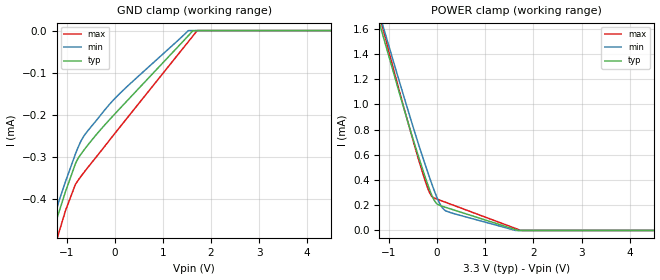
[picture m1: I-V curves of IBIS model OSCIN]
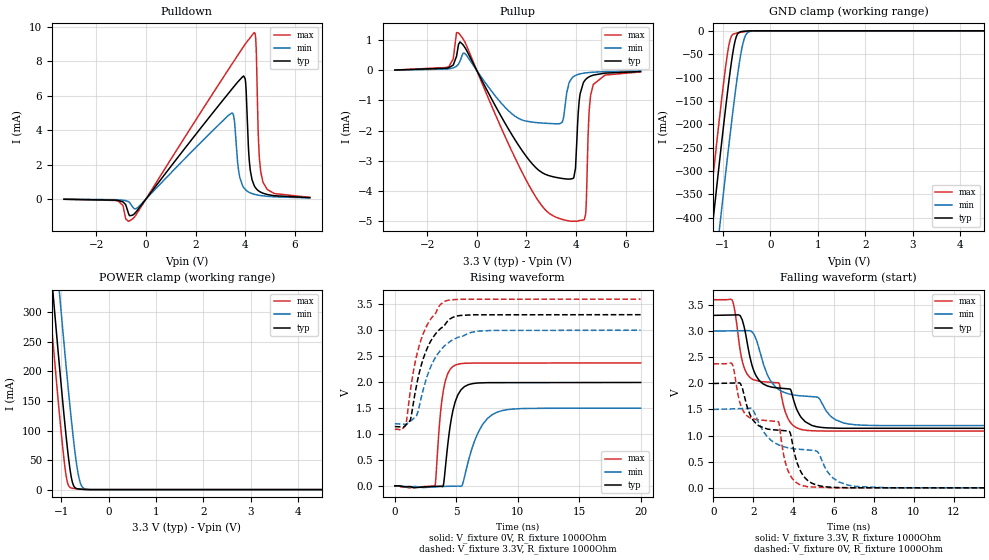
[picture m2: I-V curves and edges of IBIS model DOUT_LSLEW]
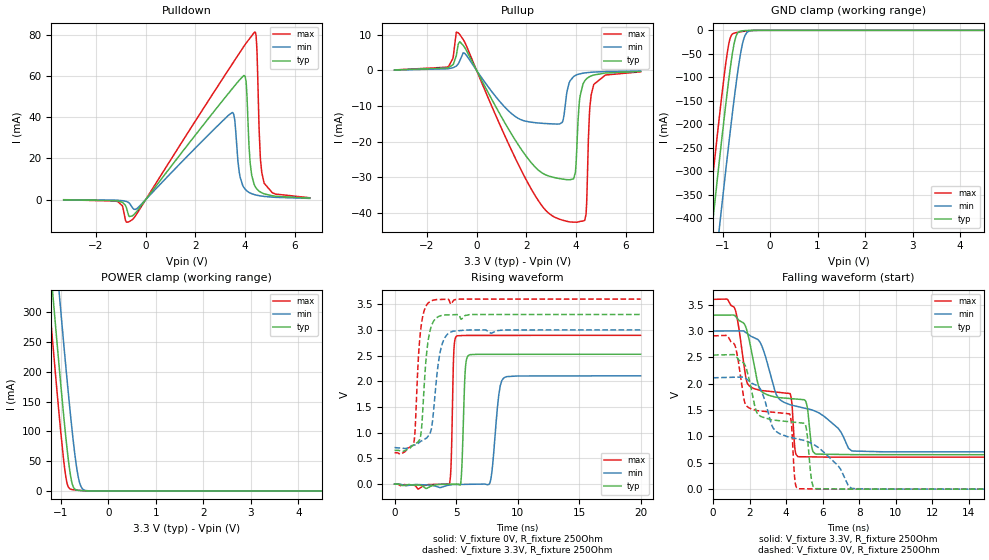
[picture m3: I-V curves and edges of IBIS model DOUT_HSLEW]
| Texas Instruments Incorporated
| LMX2615-SP Space Grade 40 MHz to 15 GHz Wideband Synthesizer with Phase
| Synchronization and JESD204B Support
[IBIS Ver]   4.1
[File name]   lmx2615.ibs
[File Rev]   1.0
[Date]   05/04/2018
[Source]   Model built from spectre simulations at:
   Texas Instruments Incorporated.
   Analog-eLab, HPA
   12500 TI Blvd
   Dallas, TX -75243
[Notes]   Revision History
| - Rev 1.0: 05/04/2018
| - C_comp although listed in numerical order of value are
|   obtained from varying PVT conditions. For PVT conditions for
|   each specific value refer the buffer description under
|   respective [Model]. IBIS model user is responsible for using
|   appropriate C_comp to simulate for Signal Integrity.
| - Notes regarding non-monotonicity of various models
|   have been reviewed and considered minor and can be ignored.
[Disclaimer]
| This model is designed as an aid for customers of Texas Instruments.
| TI and its licensors and suppliers make no warranties, either expressed
| or implied, with respect to this  model, including the warranties of
| merchantability or fitness for a particular purpose. The model is
| provided solely on an "as is" basis. The entire risk as to its quality
| and performance is with the customer.
| This model is subject to change without notice. Texas Instruments
| Incorporated is not responsible for updating this model.
[Copyright]
(C) Copyright 2018 Texas Instruments Incorporated.All rights reserved.
|  Component LMX2615W-MPR 64 pin CQFP Package
|  Part # LMX2615W-MPR
[Component]   LMX2615W-MPR
[Manufacturer]  TI
[Package]   | 64 pin CQFP Package
|   typ   min   max
R_pkg   0.05   0.04   0.06
L_pkg   1.0nH   0.8nH   1.2nH
C_pkg   0.2pF   0.16pF   0.24pF
[Pin]   signal_name   model_name   R_pin   L_pin   C_pin
1   NC   NC   NA   NA   NA
2   NC   NC   NA   NA   NA
3   FS0   INPCE   NA   NA   NA
4   FS1   INPCE   NA   NA   NA
5   CAL   INPCE   NA   NA   NA
6   GND   GND   NA   NA   NA
7   VbiasVCO   NC   NA   NA   NA
8   GND   GND   NA   NA   NA
9   NC   NC   NA   NA   NA
10   GND   GND   NA   NA   NA
11   VCCdig   POWER   NA   NA   NA
12   OSCinP   OSCIN   NA   NA   NA
13   OSCinM   OSCIN   NA   NA   NA
14   VregIN   NC   NA   NA   NA
15   FS2   INPCE   NA   NA   NA
16   FS3   INPCE   NA   NA   NA
17   FS4   INPCE   NA   NA   NA
18   FS5   INPCE   NA   NA   NA
19   FS6   INPCE   NA   NA   NA
20   FS7   INPCE   NA   NA   NA
21   VCCCP   POWER   NA   NA   NA
22   CPOUT   NC   NA   NA   NA
23   GND   GND   NA   NA   NA
24   GND   GND   NA   NA   NA
25   VCCMASH   POWER   NA   NA   NA
26   SCK   INP   NA   NA   NA
27   SDI   INP   NA   NA   NA
28   GND   GND   NA   NA   NA
29   RFOUTBM   RFOUT   NA   NA   NA
30   RFOUTBP   RFOUT   NA   NA   NA
31   GND   GND   NA   NA   NA
32   MUXOUT   DOUT   NA   NA   NA
33   NC   NC   NA   NA   NA
34   VCCBUF   POWER   NA   NA   NA
35   GND   GND   NA   NA   NA
36   RFOUTAM   RFOUT   NA   NA   NA
37   RFOUTAP   RFOUT   NA   NA   NA
38   GND   GND   NA   NA   NA
39   CSB   INP   NA   NA   NA
40   GND   GND   NA   NA   NA
41   VccVCO2   NC   NA   NA   NA
42   VbiasVCO2   NC   NA   NA   NA
43   NC   NC   NA   NA   NA
44   VrefVCO2   NC   NA   NA   NA
45   RECAL_EN   INP   NA   NA   NA
46   NC   NC   NA   NA   NA
47   NC   NC   NA   NA   NA
48   NC   NC   NA   NA   NA
49   NC   NC   NA   NA   NA
50   NC   NC   NA   NA   NA
51   GND   GND   NA   NA   NA
52   NC   NC   NA   NA   NA
53   VbiasVARAC   NC   NA   NA   NA
54   GND   GND   NA   NA   NA
55   Vtune   NC   NA   NA   NA
56   VREFVCO   NC   NA   NA   NA
57   VccVCO   NC   NA   NA   NA
58   NC   NC   NA   NA   NA
59   VregVCO   NC   NA   NA   NA
60   GND   GND   NA   NA   NA
61   GND   GND   NA   NA   NA
62   NC   NC   NA   NA   NA
63   NC   NC   NA   NA   NA
64   NC   NC   NA   NA   NA
[Diff pin]  inv_pin  vdiff  tdelay_typ  tdelay_min  tdelay_max
 12   13   0.1   NA   NA   NA
 30   29   NA   0.0s   0.0s   0.0s
 37   36   NA   0.0s   0.0s   0.0s
|  Component LMX2615W-MLS 64 pin CQFP Package
|  Part # LMX2615W-MLS
[Component]   LMX2615W-MLS
[Manufacturer]  TI
[Package]   | 64 pin CQFP Package
|   typ   min   max
R_pkg   0   0   0
L_pkg   0   0   0
C_pkg   0   0   0
[Pin]   signal_name   model_name   R_pin   L_pin   C_pin
1   NC   NC   NA   NA   NA
2   NC   NC   NA   NA   NA
3   FS0   INPCE   NA   NA   NA
4   FS1   INPCE   NA   NA   NA
5   CAL   INPCE   NA   NA   NA
6   GND   GND   NA   NA   NA
7   VbiasVCO   NC   NA   NA   NA
8   GND   GND   NA   NA   NA
9   NC   NC   NA   NA   NA
10   GND   GND   NA   NA   NA
11   VCCdig   POWER   NA   NA   NA
12   OSCinP   OSCIN   NA   NA   NA
13   OSCinM   OSCIN   NA   NA   NA
14   VregIN   NC   NA   NA   NA
15   FS2   INPCE   NA   NA   NA
16   FS3   INPCE   NA   NA   NA
17   FS4   INPCE   NA   NA   NA
18   FS5   INPCE   NA   NA   NA
19   FS6   INPCE   NA   NA   NA
20   FS7   INPCE   NA   NA   NA
21   VCCCP   POWER   NA   NA   NA
22   CPOUT   NC   NA   NA   NA
23   GND   GND   NA   NA   NA
24   GND   GND   NA   NA   NA
25   VCCMASH   POWER   NA   NA   NA
26   SCK   INP   NA   NA   NA
27   SDI   INP   NA   NA   NA
28   GND   GND   NA   NA   NA
29   RFOUTBM   RFOUT   NA   NA   NA
30   RFOUTBP   RFOUT   NA   NA   NA
31   GND   GND   NA   NA   NA
32   MUXOUT   DOUT   NA   NA   NA
33   NC   NC   NA   NA   NA
34   VCCBUF   POWER   NA   NA   NA
35   GND   GND   NA   NA   NA
36   RFOUTAM   RFOUT   NA   NA   NA
37   RFOUTAP   RFOUT   NA   NA   NA
38   GND   GND   NA   NA   NA
39   CSB   INP   NA   NA   NA
40   GND   GND   NA   NA   NA
41   VccVCO2   NC   NA   NA   NA
42   VbiasVCO2   NC   NA   NA   NA
43   NC   NC   NA   NA   NA
44   VrefVCO2   NC   NA   NA   NA
45   RECAL_EN   INP   NA   NA   NA
46   NC   NC   NA   NA   NA
47   NC   NC   NA   NA   NA
48   NC   NC   NA   NA   NA
49   NC   NC   NA   NA   NA
50   NC   NC   NA   NA   NA
51   GND   GND   NA   NA   NA
52   NC   NC   NA   NA   NA
53   VbiasVARAC   NC   NA   NA   NA
54   GND   GND   NA   NA   NA
55   Vtune   NC   NA   NA   NA
56   VREFVCO   NC   NA   NA   NA
57   VccVCO   NC   NA   NA   NA
58   NC   NC   NA   NA   NA
59   VregVCO   NC   NA   NA   NA
60   GND   GND   NA   NA   NA
61   GND   GND   NA   NA   NA
62   NC   NC   NA   NA   NA
63   NC   NC   NA   NA   NA
64   NC   NC   NA   NA   NA
[Diff pin]  inv_pin  vdiff  tdelay_typ  tdelay_min  tdelay_max
 12   13   0.1   NA   NA   NA
 30   29   NA   0.0s   0.0s   0.0s
 37   36   NA   0.0s   0.0s   0.0s
|   Model Selectors
[Model Selector] DOUT
DOUT_LSLEW   3.3V OUTPUT, low slew rate
DOUT_HSLEW   3.3V OUTPUT, high slew rate
| Models and submodels in the file (6): OSCIN (Input), DOUT_LSLEW (3-state), DOUT_HSLEW (3-state), INP (Input), INPCE (Input), RFOUT (Open_drain)
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|   Model OSCIN
[Model]   OSCIN
Model_type   Input
Vinl = .4
Vinh = 1.8
|   typ   min   max
C_comp   0.219p   0.215p   0.221p
[Voltage Range]   3.3   3.15   3.45
[Temperature Range]   27   125   -40
[Power Clamp Reference]   3.3   3.15   3.45
[GND Clamp Reference]   0   0   0
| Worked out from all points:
|   GND clamp passes 1 mA (typ) near -2.28 V on its own axis
|   POWER clamp passes 1 mA (typ) near -0.72 V on its own axis
[GND Clamp]
|   Voltage   I(typ)   I(min)   I(max)
-3.3V     -1.834mA   -1.951mA   -1.829mA
-1.508V   -565uA     -564.9uA   -620uA
-1.31V    -487.7uA   -467.1uA   -540.3uA
-1.152V   -429.5uA   -403.3uA   -477.7uA
-1.023V   -383.4uA   -359.6uA   -428.6uA
-815.1mV  -316.6uA   -293.4uA   -365.7uA
-607.2mV  -279.5uA   -245.5uA   -332.8uA
85.8mV    -188.1uA   -152.1uA   -232.8uA
1.531V    -12.08uA   -44.6nA    -26.36uA
1.62V     -735.5nA   0A         -13.62uA
1.729V    0A         0A         0A
6.6V      0A         0A         0A
[POWER Clamp]
|   Voltage   I(typ)   I(min)   I(max)
-3.3V     5.966mA    6.361mA    6.077mA
-1.231V   1.684mA    1.757mA    1.748mA
-815.1mV  1.129mA    1.218mA    1.146mA
-409.2mV  611.5uA    709.5uA    592.2uA
-181.5mV  349.1uA    446uA      320.6uA
-112.2mV  280.1uA    369.9uA    271.2uA
-23.1mV   218uA      278.7uA    251.5uA
105.6mV   191.7uA    180.2uA    233.1uA
184.8mV   182uA      154.2uA    221.8uA
1.63V     6.809uA    0A         15.72uA
1.729V    0A         0A         1.069uA
6.6V      0A         0A         0A
|   Model DOUT_LSLEW
[Model]   DOUT_LSLEW
Model_type   3-state
Polarity   Non-Inverting
Vmeas = 1.65
Vref = 3.3
Cref = 1pF
Rref = 1000
|   typ   min   max
|   (nom PVT)   (fast PVT)   (slow PVT)
C_comp   1.019p   0.968p   1.051p
[Voltage Range]   3.3   3   3.6
[Temperature Range]   27   125   -40
[Pullup Reference]   3.3   3   3.6
[Pulldown Reference]   0   0   0
[Power Clamp Reference]   3.3   3   3.6
[GND Clamp Reference]   0   0   0
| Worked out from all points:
|   slope of the pulldown table from 0 to 0.495 V, typ, clamps not added: 528 ohm
|   slope of the pullup table from 0 to 0.495 V, typ, clamps not added: 627 ohm
|   GND clamp passes 1 mA (typ) near -0.57 V on its own axis
|   POWER clamp passes 1 mA (typ) near -0.63 V on its own axis
|   falling waveform, V_fixture 3.3V, R_fixture 1000Ohm: 20-80 % time 2.45ns typ, 3.22ns min, 2.31ns max; typ from 3.3 V to 1.14 V
|   rising waveform, V_fixture 0V, R_fixture 1000Ohm: 20-80 % time 749ps typ, 1.4ns min, 569ps max; typ from 0 V to 1.99 V
|   rising waveform, V_fixture 3.3V, R_fixture 1000Ohm: 20-80 % time 1.63ns typ, 1.79ns min, 1.49ns max; typ from 1.14 V to 3.3 V
|   falling waveform, V_fixture 0V, R_fixture 1000Ohm: 20-80 % time 2.61ns typ, 3.39ns min, 2.43ns max; typ from 2 V to 0 V
[Pulldown]
|   Voltage   I(typ)   I(min)   I(max)
-3.3V     -11.43uA   -7.802uA   -12.1uA
-537.9mV  -936.6uA   -451.7uA   -1.153mA
3.462V    6.382mA    4.997mA    7.828mA
3.759V    6.891mA    1.418mA    8.479mA
3.937V    7.142mA    671.1uA    8.867mA
4.016V    6.747mA    535.7uA    9.031mA
4.165V    2.21mA     385.6uA    9.304mA
4.372V    751.3uA    275.1uA    9.665mA
4.442V    605.9uA    250.9uA    8.713mA
4.561V    452.6uA    217.8uA    2.597mA
4.709V    342.4uA    186.9uA    1.005mA
6.6V      81.82uA    66.05uA    100.7uA
[GND Clamp]
|   Voltage   I(typ)   I(min)   I(max)
-3.3V     -2.452A    -2.589A    -2.364A
-1.439V   -627.2mA   -770.9mA   -533mA
-1.27V    -466.7mA   -610.7mA   -372.2mA
-1.211V   -410.7mA   -554.6mA   -316.2mA
-1.073V   -282mA     -425.3mA   -188.4mA
-1.033V   -246mA     -388.8mA   -153.2mA
-874.5mV  -109.2mA   -246.3mA   -31.62mA
-765.6mV  -33.07mA   -153.9mA   -6.398mA
-696.3mV  -7.92mA    -99.78mA   -4.642mA
-577.5mV  -1.073mA   -27.36mA   -2.516mA
-419.1mV  -88.15uA   -1.084mA   -769.1uA
6.6V      0A         0A         0A
[Pullup]
|   Voltage   I(typ)   I(min)   I(max)
-3.3V     12.07uA    9.347uA    12.51uA
-1.132V   89.8uA     52.94uA    125.7uA
-735.9mV  862.4uA    206.3uA    1.249mA
2.234V    -3.109mA   -1.72mA    -4.015mA
3.432V    -3.594mA   -1.729mA   -4.955mA
3.858V    -3.601mA   -234.1uA   -5.021mA
3.977V    -3.257mA   -167uA     -5.022mA
4.145V    -883.9uA   -117.5uA   -4.995mA
4.382V    -304.1uA   -82.23uA   -4.8mA
4.521V    -215.1uA   -69.84uA   -1.435mA
4.699V    -155.4uA   -58.43uA   -464.3uA
6.6V      -38.28uA   -21.08uA   -49.46uA
[POWER Clamp]
|   Voltage   I(typ)   I(min)   I(max)
-3.3V     2.408A     2.526A     2.331A
-1.389V   536.7mA    662mA      454.1mA
-1.231V   386.9mA    512.5mA    303.9mA
-1.171V   331.5mA    457.1mA    248.6mA
-1.053V   223.1mA    347.7mA    141.4mA
-1.013V   188mA      311.9mA    107.5mA
-894.3mV  88.96mA    207.3mA    22.7mA
-795.3mV  24.72mA    125.6mA    2.896mA
-735.9mV  6.329mA    81.34mA    1.968mA
-636.9mV  1.065mA    24.47mA    1.107mA
-478.5mV  181.4uA    709.5uA    176.1uA
6.6V      0A         0A         0A
[Ramp]
R_load = 1000
|   typ   min   max
dV/dt_r   1.19558/7.49454e-10   0.89825/1.40115e-09   1.4217/5.69081e-10
dV/dt_f   1.29663/2.44804e-09   1.08511/3.20365e-09   1.50804/2.31143e-09
[Falling Waveform]
V_fixture = 3.3V
V_fixture_min = 3V
V_fixture_max = 3.6V
R_fixture = 1000Ohm
C_fixture = 0F
|   Time   V(typ)   V(min)   V(max)
0s        3.3V       3V         3.6V
928.8ps   3.307V     3.005V     3.597V
1.34ns    3.295V     3.007V     2.629V
1.669ns   2.822V     3.008V     2.186V
2.149ns   2.133V     2.83V      2.054V
3.27ns    1.91V      1.88V      2.009V
3.726ns   1.894V     1.801V     1.326V
4.301ns   1.398V     1.763V     1.126V
7.116ns   1.14V      1.206V     1.087V
20ns      1.139V     1.191V     1.087V
[Rising Waveform]
V_fixture = 0V
V_fixture_min = 0V
V_fixture_max = 0V
R_fixture = 1000Ohm
C_fixture = 0F
|   Time   V(typ)   V(min)   V(max)
0s        108.1nV    2.108uV    192.6nV
3.27ns    -11.22mV   -20.47mV   -5.748mV
3.646ns   -8.576mV   -15.22mV   1.222V
3.959ns   25.78mV    -12.06mV   1.856V
4.475ns   1.109V     -8.854mV   2.236V
4.982ns   1.663V     -6.554mV   2.334V
5.506ns   1.879V     28.86mV    2.359V
7.116ns   1.986V     1.173V     2.367V
8.316ns   1.989V     1.42V      2.368V
20ns      1.993V     1.497V     2.369V
[Rising Waveform]
V_fixture = 3.3V
V_fixture_min = 3V
V_fixture_max = 3.6V
R_fixture = 1000Ohm
C_fixture = 0F
|   Time   V(typ)   V(min)   V(max)
0s        1.143V     1.197V     1.09V
895.1ps   1.171V     1.19V      1.179V
1.276ns   1.282V     1.246V     1.854V
1.754ns   1.92V      1.348V     2.487V
2.149ns   2.324V     1.699V     2.83V
2.7ns     2.688V     2.161V     3.13V
3.959ns   3.069V     2.678V     3.546V
4.913ns   3.265V     2.838V     3.592V
6.751ns   3.297V     2.982V     3.597V
20ns      3.3V       3V         3.6V
[Falling Waveform]
|Gnd
V_fixture = 0V
V_fixture_min = 0V
V_fixture_max = 0V
R_fixture = 1000Ohm
C_fixture = 0F
|   Time   V(typ)   V(min)   V(max)
0s        1.997V     1.5V       2.373V
928.8ps   2.005V     1.511V     2.376V
1.361ns   1.988V     1.517V     1.589V
1.669ns   1.573V     1.52V      1.381V
2.149ns   1.222V     1.348V     1.305V
3.248ns   1.103V     824mV      1.268V
3.726ns   1.089V     767mV      330.1mV
4.499ns   228.9mV    731.5mV    37.34mV
7.116ns   2.047mV    26.75mV    744.9uV
20ns      -35.77uV   -26.42uV   -32.15uV
|   Model DOUT_HSLEW
[Model]   DOUT_HSLEW
Model_type   3-state
Polarity   Non-Inverting
Vmeas = 1.65
Vref = 3.3
Cref = 1pF
Rref = 250
|   typ   min   max
|   (nom PVT)   (fast PVT)   (slow PVT)
C_comp   1.019p   0.968p   1.051p
[Voltage Range]   3.3   3   3.6
[Temperature Range]   27   125   -40
[Pullup Reference]   3.3   3   3.6
[Pulldown Reference]   -0   0   -0
[Power Clamp Reference]   3.3   3   3.6
[GND Clamp Reference]   0   0   0
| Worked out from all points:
|   slope of the pulldown table from 0 to 0.495 V, typ, clamps not added: 63 ohm
|   slope of the pullup table from 0 to 0.495 V, typ, clamps not added: 74.7 ohm
|   GND clamp passes 1 mA (typ) near -0.57 V on its own axis
|   POWER clamp passes 1 mA (typ) near -0.63 V on its own axis
|   falling waveform, V_fixture 3.3V, R_fixture 250Ohm: 20-80 % time 3.26ns typ, 3.97ns min, 2.96ns max; typ from 3.3 V to 0.654 V
|   rising waveform, V_fixture 0V, R_fixture 250Ohm: 20-80 % time 206ps typ, 459ps min, 158ps max; typ from 0 V to 2.53 V
|   rising waveform, V_fixture 3.3V, R_fixture 250Ohm: 20-80 % time 493ps typ, 630ps min, 422ps max; typ from 0.657 V to 3.3 V
|   falling waveform, V_fixture 0V, R_fixture 250Ohm: 20-80 % time 3.28ns typ, 4.07ns min, 2.97ns max; typ from 2.54 V to 0 V
[Pulldown]
|   Voltage   I(typ)   I(min)   I(max)
-3.3V     -97.31uA   -66.38uA   -103.1uA
-537.9mV  -7.903mA   -3.884mA   -9.711mA
3.482V    53.83mA    42.24mA    65.82mA
3.759V    57.85mA    13.57mA    70.91mA
3.957V    60.23mA    5.716mA    74.52mA
4.046V    56.01mA    4.447mA    76.07mA
4.204V    17.43mA    3.161mA    78.53mA
4.392V    6.6mA      2.34mA     81.3mA
4.471V    5.142mA    2.107mA    73.28mA
4.61V     3.684mA    1.794mA    20.61mA
4.759V    2.815mA    1.546mA    8.205mA
6.6V      703.7uA    565.4uA    872.6uA
[GND Clamp]
|   Voltage   I(typ)   I(min)   I(max)
-3.3V     -2.452A    -2.589A    -2.364A
-1.439V   -627.2mA   -770.9mA   -533mA
-1.27V    -466.7mA   -610.7mA   -372.2mA
-1.211V   -410.7mA   -554.6mA   -316.2mA
-1.073V   -282mA     -425.3mA   -188.4mA
-1.033V   -246mA     -388.8mA   -153.2mA
-874.5mV  -109.2mA   -246.3mA   -31.62mA
-765.6mV  -33.07mA   -153.9mA   -6.398mA
-696.3mV  -7.92mA    -99.78mA   -4.642mA
-577.5mV  -1.073mA   -27.36mA   -2.516mA
-419.1mV  -88.15uA   -1.084mA   -769.1uA
6.6V      0A         0A         0A
[Pullup]
|   Voltage   I(typ)   I(min)   I(max)
-3.3V     103.2uA    82.1uA     106.6uA
-1.132V   773.6uA    462.9uA    1.092mA
-735.9mV  7.422mA    1.805mA    10.54mA
2.452V    -27.83mA   -14.78mA   -36.26mA
3.442V    -30.54mA   -14.66mA   -42.06mA
3.719V    -30.74mA   -3.65mA    -42.54mA
4.006V    -25.89mA   -1.343mA   -42.67mA
4.155V    -7.744mA   -993.3uA   -42.46mA
4.402V    -2.541mA   -687.5uA   -40.52mA
4.541V    -1.805mA   -585.3uA   -12.25mA
4.719V    -1.308mA   -490.8uA   -3.945mA
6.6V      -327.2uA   -179.6uA   -424.3uA
[POWER Clamp]
|   Voltage   I(typ)   I(min)   I(max)
-3.3V     2.408A     2.526A     2.331A
-1.389V   536.7mA    662mA      454.1mA
-1.231V   386.9mA    512.5mA    303.9mA
-1.171V   331.5mA    457.1mA    248.6mA
-1.053V   223.1mA    347.7mA    141.4mA
-1.013V   188mA      311.9mA    107.5mA
-894.3mV  88.96mA    207.3mA    22.7mA
-795.3mV  24.72mA    125.6mA    2.896mA
-735.9mV  6.329mA    81.34mA    1.968mA
-636.9mV  1.065mA    24.47mA    1.107mA
-478.5mV  181.4uA    709.5uA    176.1uA
6.6V      0A         0A         0A
[Ramp]
R_load = 250
|   typ   min   max
dV/dt_r   1.51618/2.06185e-10   1.26405/4.58899e-10   1.73655/1.57782e-10
dV/dt_f   1.58787/3.26139e-09   1.37589/3.97049e-09   1.79585/2.95886e-09
[Falling Waveform]
V_fixture = 3.3V
V_fixture_min = 3V
V_fixture_max = 3.6V
R_fixture = 250Ohm
C_fixture = 0F
|   Time   V(typ)   V(min)   V(max)
0s        3.3V       3V         3.6V
1.185ns   3.294V     3.001V     3.431V
1.908ns   2.931V     2.943V     1.99V
2.549ns   1.9V       2.799V     1.876V
4.216ns   1.719V     1.603V     1.814V
4.638ns   1.707V     1.567V     619mV
5.103ns   1.638V     1.529V     613.4mV
5.646ns   664.9mV    1.47V      611mV
7.635ns   655.2mV    723.3mV    607.1mV
20ns      653.6mV    706.9mV    606.9mV
[Rising Waveform]
V_fixture = 0V
V_fixture_min = 0V
V_fixture_max = 0V
R_fixture = 250Ohm
C_fixture = 0F
|   Time   V(typ)   V(min)   V(max)
0s        15.55nV    -303.8nV   26.96nV
4.451ns   -2.775mV   -19.97mV   -9.847mV
4.803ns   -1.285mV   -8.54mV    2.496V
5.03ns    -326.5uV   -7.751mV   2.877V
5.391ns   39.94mV    -6.492mV   2.889V
5.732ns   2.159V     -5.305mV   2.892V
6.045ns   2.51V      -4.216mV   2.892V
7.784ns   2.525V     48.56mV    2.893V
8.866ns   2.525V     2.063V     2.893V
20ns      2.527V     2.107V     2.894V
[Rising Waveform]
V_fixture = 3.3V
V_fixture_min = 3V
V_fixture_max = 3.6V
R_fixture = 250Ohm
C_fixture = 0F
|   Time   V(typ)   V(min)   V(max)
0s        656.7mV    711.1mV    609.3mV
1.559ns   764.3mV    754.9mV    804.1mV
1.665ns   780.4mV    762.9mV    1.022V
2.04ns    867.8mV    816.4mV    2.794V
2.208ns   1.114V     842.3mV    3.154V
2.628ns   2.594V     900.7mV    3.488V
2.926ns   3.021V     1.016V     3.559V
3.68ns    3.269V     2.539V     3.592V
4.483ns   3.294V     2.948V     3.547V
20ns      3.3V       3V         3.6V
[Falling Waveform]
|Gnd
V_fixture = 0V
V_fixture_min = 0V
V_fixture_max = 0V
R_fixture = 250Ohm
C_fixture = 0F
|   Time   V(typ)   V(min)   V(max)
0s        2.543V     2.112V     2.907V
1.185ns   2.542V     2.123V     2.739V
1.856ns   2.245V     2.084V     1.571V
2.411ns   1.443V     1.966V     1.49V
4.195ns   1.279V     986.7mV    1.429V
4.638ns   1.263V     951.7mV    11.81mV
5.073ns   1.202V     915.5mV    6.309mV
5.646ns   9.5mV      817mV      3.978mV
7.635ns   1.017mV    12.52mV    343.9uV
20ns      -36.48uV   -53.2uV    -27.43uV
